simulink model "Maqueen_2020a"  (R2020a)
settings: Solver=VariableStepAuto  StartTime=0.0  StopTime=2  RelTol=1e-3
model workspace: external: MAT-File (data not in the file)
undefined symbols (not defined in the file or in its folder): deg, kg, m, mm, N, rad, s, smiData, X, Y, Z
libraries: sm_lib x459, fl_lib x12, nesl_utility x10
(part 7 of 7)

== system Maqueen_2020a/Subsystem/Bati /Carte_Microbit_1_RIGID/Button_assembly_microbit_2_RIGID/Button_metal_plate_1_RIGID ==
  ReferenceFrame : sm_lib/Frames and Transforms/Reference Frame
  Solid : sm_lib/Body Elements/File Solid  ExtGeomFileName=Button metal plate_Defaut_sldprt.STL  UnitType=Custom  ExtGeomFileUnits=mm  StepReaderType=HEX  ExportConvexHullGeometry=off  InertiaType=Custom  Mass=smiData.Solid(25).mass  MassUnits=kg  CenterOfMass=smiData.Solid(25).CoM  CenterOfMassUnits=mm  MomentsOfInertia=smiData.Solid(25).MoI  MomentsOfInertiaUnits=kg*mm^2  ProductsOfInertia=smiData.Solid(25).PoI  ProductsOfInertiaUnits=kg*mm^2  BasedOnType=Density  Density=1000  DensityUnits=kg/m^3  DoExposeReferenceFrame=on  SerializedFrames=<Frames/>  GraphicType=FromGeometry  MarkerShape=Sphere  MarkerSize=10  GraphicVisPropType=SimpleVisualProperties  GraphicDiffuseColor=smiData.Solid(25).color  GraphicSpecularColor=[0.5 0.5 0.5 1.0]  GraphicAmbientColor=[0.15 0.15 0.15 1.0]  GraphicEmissiveColor=[0.0 0.0 0.0 1.0]  GraphicShininess=75  GraphicOpacity=smiData.Solid(25).opacity
  F : PMIOPort  Side=Left
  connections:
  ReferenceFrame/RConn1 -- Solid/RConn1 -- F/RConn1

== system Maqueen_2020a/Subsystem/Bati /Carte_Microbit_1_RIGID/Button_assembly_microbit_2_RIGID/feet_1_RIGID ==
  ReferenceFrame : sm_lib/Frames and Transforms/Reference Frame
  Solid : sm_lib/Body Elements/File Solid  ExtGeomFileName=feet_Defaut_sldprt.STL  UnitType=Custom  ExtGeomFileUnits=mm  StepReaderType=HEX  ExportConvexHullGeometry=off  InertiaType=Custom  Mass=smiData.Solid(24).mass  MassUnits=kg  CenterOfMass=smiData.Solid(24).CoM  CenterOfMassUnits=mm  MomentsOfInertia=smiData.Solid(24).MoI  MomentsOfInertiaUnits=kg*mm^2  ProductsOfInertia=smiData.Solid(24).PoI  ProductsOfInertiaUnits=kg*mm^2  BasedOnType=Density  Density=1000  DensityUnits=kg/m^3  DoExposeReferenceFrame=on  SerializedFrames=<Frames/>  GraphicType=FromGeometry  MarkerShape=Sphere  MarkerSize=10  GraphicVisPropType=SimpleVisualProperties  GraphicDiffuseColor=smiData.Solid(24).color  GraphicSpecularColor=[0.5 0.5 0.5 1.0]  GraphicAmbientColor=[0.15 0.15 0.15 1.0]  GraphicEmissiveColor=[0.0 0.0 0.0 1.0]  GraphicShininess=75  GraphicOpacity=smiData.Solid(24).opacity
  F : PMIOPort  Side=Left
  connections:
  ReferenceFrame/RConn1 -- Solid/RConn1 -- F/RConn1

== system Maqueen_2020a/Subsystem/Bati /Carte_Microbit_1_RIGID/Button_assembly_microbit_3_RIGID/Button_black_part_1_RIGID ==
  ReferenceFrame : sm_lib/Frames and Transforms/Reference Frame
  Solid : sm_lib/Body Elements/File Solid  ExtGeomFileName=Button black part_Defaut_sldprt.STL  UnitType=Custom  ExtGeomFileUnits=mm  StepReaderType=HEX  ExportConvexHullGeometry=off  InertiaType=Custom  Mass=smiData.Solid(23).mass  MassUnits=kg  CenterOfMass=smiData.Solid(23).CoM  CenterOfMassUnits=mm  MomentsOfInertia=smiData.Solid(23).MoI  MomentsOfInertiaUnits=kg*mm^2  ProductsOfInertia=smiData.Solid(23).PoI  ProductsOfInertiaUnits=kg*mm^2  BasedOnType=Density  Density=1000  DensityUnits=kg/m^3  DoExposeReferenceFrame=on  SerializedFrames=<Frames/>  GraphicType=FromGeometry  MarkerShape=Sphere  MarkerSize=10  GraphicVisPropType=SimpleVisualProperties  GraphicDiffuseColor=smiData.Solid(23).color  GraphicSpecularColor=[0.5 0.5 0.5 1.0]  GraphicAmbientColor=[0.15 0.15 0.15 1.0]  GraphicEmissiveColor=[0.0 0.0 0.0 1.0]  GraphicShininess=75  GraphicOpacity=smiData.Solid(23).opacity
  F : PMIOPort  Side=Left
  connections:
  ReferenceFrame/RConn1 -- Solid/RConn1 -- F/RConn1

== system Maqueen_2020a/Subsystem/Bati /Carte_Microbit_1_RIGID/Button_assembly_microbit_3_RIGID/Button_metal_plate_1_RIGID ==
  ReferenceFrame : sm_lib/Frames and Transforms/Reference Frame
  Solid : sm_lib/Body Elements/File Solid  ExtGeomFileName=Button metal plate_Defaut_sldprt.STL  UnitType=Custom  ExtGeomFileUnits=mm  StepReaderType=HEX  ExportConvexHullGeometry=off  InertiaType=Custom  Mass=smiData.Solid(25).mass  MassUnits=kg  CenterOfMass=smiData.Solid(25).CoM  CenterOfMassUnits=mm  MomentsOfInertia=smiData.Solid(25).MoI  MomentsOfInertiaUnits=kg*mm^2  ProductsOfInertia=smiData.Solid(25).PoI  ProductsOfInertiaUnits=kg*mm^2  BasedOnType=Density  Density=1000  DensityUnits=kg/m^3  DoExposeReferenceFrame=on  SerializedFrames=<Frames/>  GraphicType=FromGeometry  MarkerShape=Sphere  MarkerSize=10  GraphicVisPropType=SimpleVisualProperties  GraphicDiffuseColor=smiData.Solid(25).color  GraphicSpecularColor=[0.5 0.5 0.5 1.0]  GraphicAmbientColor=[0.15 0.15 0.15 1.0]  GraphicEmissiveColor=[0.0 0.0 0.0 1.0]  GraphicShininess=75  GraphicOpacity=smiData.Solid(25).opacity
  F : PMIOPort  Side=Left
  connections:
  ReferenceFrame/RConn1 -- Solid/RConn1 -- F/RConn1

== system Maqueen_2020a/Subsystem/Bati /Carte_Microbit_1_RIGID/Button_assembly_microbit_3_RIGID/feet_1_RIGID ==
  ReferenceFrame : sm_lib/Frames and Transforms/Reference Frame
  Solid : sm_lib/Body Elements/File Solid  ExtGeomFileName=feet_Defaut_sldprt.STL  UnitType=Custom  ExtGeomFileUnits=mm  StepReaderType=HEX  ExportConvexHullGeometry=off  InertiaType=Custom  Mass=smiData.Solid(24).mass  MassUnits=kg  CenterOfMass=smiData.Solid(24).CoM  CenterOfMassUnits=mm  MomentsOfInertia=smiData.Solid(24).MoI  MomentsOfInertiaUnits=kg*mm^2  ProductsOfInertia=smiData.Solid(24).PoI  ProductsOfInertiaUnits=kg*mm^2  BasedOnType=Density  Density=1000  DensityUnits=kg/m^3  DoExposeReferenceFrame=on  SerializedFrames=<Frames/>  GraphicType=FromGeometry  MarkerShape=Sphere  MarkerSize=10  GraphicVisPropType=SimpleVisualProperties  GraphicDiffuseColor=smiData.Solid(24).color  GraphicSpecularColor=[0.5 0.5 0.5 1.0]  GraphicAmbientColor=[0.15 0.15 0.15 1.0]  GraphicEmissiveColor=[0.0 0.0 0.0 1.0]  GraphicShininess=75  GraphicOpacity=smiData.Solid(24).opacity
  F : PMIOPort  Side=Left
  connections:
  ReferenceFrame/RConn1 -- Solid/RConn1 -- F/RConn1
